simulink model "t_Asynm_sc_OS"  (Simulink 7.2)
settings: Solver=ode3  StartTime=0.0  StopTime=0.5  FixedStep=10e-6  MaxStep=1e-4  RelTol=1e-4  AbsTol=1e-4
libraries: simulink x1

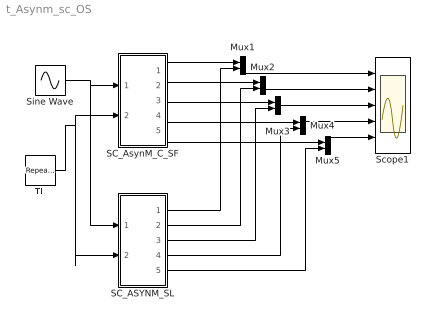
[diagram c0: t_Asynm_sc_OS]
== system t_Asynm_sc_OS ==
  Mux{1..5} (5 alike) : Mux  Inputs=2
  SC_ASYNM_SL : Subsystem  mask(SC_ASYN_MOTOR){rs=0.087, Lls=0.8e-3, rr=0.228, Llr=0.8e-3, Lm=34.7e-3, P=4, J=0.8, D=0.1, omm0=0}
      mask prompts: rs "Stator Resistance"; Lls "Stator Leakage Inductance"; rr "Rotor Resistance"; Llr "Rotor Leakage Inductance"; Lm "Magnetising Inductance"; P "Number of Poles"; J "Moment of Inertia"; D "Damping Coefficient"; omm0 "initial ang. speed"
      mask help: Open source Squirrel cage Asyn. MOTOR modeled in Simulink Blocks Input Vector u: u[0,1,2]= Three phase stator Voltages u[3]= Load Torque Output Vector y: y[0,1,2]= Three phase stator Currents y[3]= Te y[4]= Ang. Velocity W Parameter Vector p: p[0]= Rs p[1]= Ls p[2]= Rr p[3]= Lr p[4]= LM p[5]= Number of Poles P p[6]= Moment of Inertia J p[7]= Damp. Coef. D p[8]= Initial Ang. Velocity W0 You can pause the simulation during running, change the Parameters you want and continue the Simulation
  SC_AsynM_C_SF : Subsystem  mask(SC_ASYN_MOTOR){RS=0.087, LS=0.8e-3, RR=0.228, LR=0.8e-3, LM=34.7e-3, P=4, J=0.8, D=0.1, W0=0}
      mask prompts: RS "Stator Resistance"; LS "Stator Leakage Inductance"; RR "Rotor Resistance"; LR "Rotor Leakage Inductance"; LM "Magnetising Inductance"; P "Number of Poles"; J "Moment of Inertia"; D "Damping Coefficient"; W0 "initial ang. speed"
      mask help: Open source Squirrel cage Asyn. MOTOR modeled as Simulink C-S-Function Block Input Vector u: u[0,1,2]= Three phase stator Voltages u[3]= Load Torque Output Vector y: y[0,1,2]= Three phase stator Currents y[3]= Te y[4]= Ang. Velocity W Parameter Vector p: p[0]= Rs p[1]= Ls p[2]= Rr p[3]= Lr p[4]= LM p[5]= Number of Poles P p[6]= Moment of Inertia J p[7]= Damp. Coef. D p[8]= Initial Ang. Velocity W0 You can pause the simulation during running, change the Parameters you want and continue the Simulation
  Scope1 : Scope  NumInputPorts=5
  Sine Wave : Sin  Amplitude=400*sqrt(2)  Frequency=50*2*pi  Phase=[0, -2*pi/3, -4*pi/3]  SampleTime=0
  TL : simulink/Sources/Repeating Sequence  SystemSampleTime=-1  rep_seq_t="[0      0.2     0.201      0.4    0.401     1 ]"  rep_seq_y="[0       0       1000     1000   -1000   -1000]"
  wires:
  Sine Wave/1 -> SC_AsynM_C_SF/1(Vabc), SC_ASYNM_SL/1(Vabc)
  TL/1 -> SC_AsynM_C_SF/2(TL), SC_ASYNM_SL/2(Tl)
  Mux1/1 -> Scope1/1
  Mux2/1 -> Scope1/2
  Mux3/1 -> Scope1/3
  Mux4/1 -> Scope1/4
  Mux5/1 -> Scope1/5
  SC_ASYNM_SL/1(ia) -> Mux1/2
  SC_ASYNM_SL/2(ib) -> Mux2/2
  SC_ASYNM_SL/3(ic) -> Mux3/2
  SC_AsynM_C_SF/5(W) -> Mux5/1
  SC_AsynM_C_SF/1(iA) -> Mux1/1
  SC_AsynM_C_SF/2(iB) -> Mux2/1
  SC_AsynM_C_SF/3(iC) -> Mux3/1
  SC_AsynM_C_SF/4(TE) -> Mux4/1
  SC_ASYNM_SL/4(Te) -> Mux4/2
  SC_ASYNM_SL/5(w) -> Mux5/2

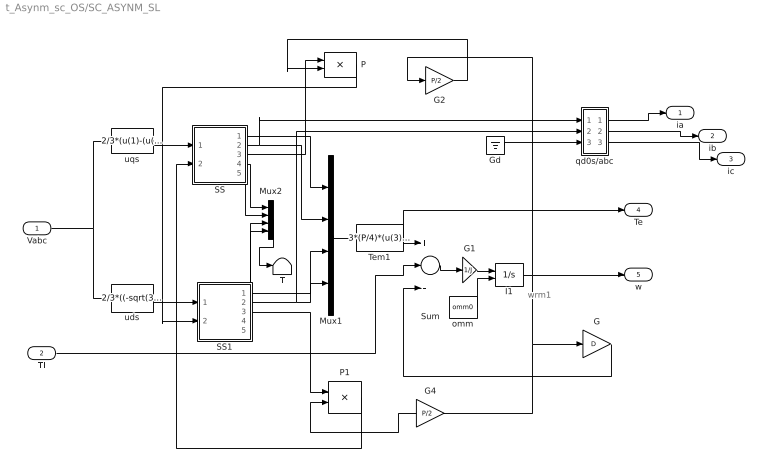
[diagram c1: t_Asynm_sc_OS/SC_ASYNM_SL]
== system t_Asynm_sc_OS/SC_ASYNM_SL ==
  note: wrm1
  Vabc : Inport
  Tl : Inport  Port=2
  G : Gain  Gain=D
  G1 : Gain  Gain=1/J
  G2 : Gain  Gain=P/2
  G4 : Gain  Gain=P/2
  Gd : Ground
  I1 : Integrator  InitialConditionSource=external
  Mux1 : Mux
  Mux2 : Mux
  P : Product
  P1 : Product
  SS : Subsystem
  SS1 : Subsystem
  Sum : Sum  Inputs=+--
  T : Terminator
  Tem1 : Fcn  Expr=3*(P/4)*(u(3)*u(2)-u(1)*u(4))
  omm : Constant  Value=omm0
  qd0s/abc : Subsystem
  uds : Fcn  Expr=2/3*((-sqrt(3)/2)*u(2)+(sqrt(3)/2)*u(3))
  uqs : Fcn  Expr=2/3*(u(1)-(u(2)/2)-(u(3)/2))
  ia : Outport
  ib : Outport  Port=2
  ic : Outport  Port=3
  Te : Outport  Port=4
  w : Outport  Port=5
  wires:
  Gd/1 -> qd0s/abc/3(0)
  SS1/1(psids) -> Mux1/3
  SS1/2(ids) -> qd0s/abc/2(d), Mux1/4
  SS1/3(psidr) -> P1/1
  SS/3(psiqr) -> P/1
  SS/1(psiqs) -> Mux1/1
  Tl/1 -> Sum/2
  Tem1/1 -> Te/1, Sum/1
  SS/2(iqs) -> qd0s/abc/1(q), Mux1/2
  G/1 -> Sum/3
  I1/1 -> w/1, G2/1, G4/1, G/1
  P/1 -> SS1/2(wr*psiqr)
  P1/1 -> SS/2(wr*psidr)
  Vabc/1 -> uds/1, uqs/1
  uds/1 -> SS1/1(uds)
  uqs/1 -> SS/1(uqs)
  G4/1 -> P1/2
  G2/1 -> P/2
  Sum/1 -> G1/1
  Mux1/1 -> Tem1/1
  SS/4(iqr) -> Mux2/1
  SS/5(psiqm) -> Mux2/2
  SS1/4(idr) -> Mux2/3
  SS1/5(psidm) -> Mux2/4
  Mux2/1 -> T/1
  G1/1 -> I1/1
  omm/1 -> I1/2
  qd0s/abc/1(a) -> ia/1
  qd0s/abc/2(b) -> ib/1
  qd0s/abc/3(c) -> ic/1

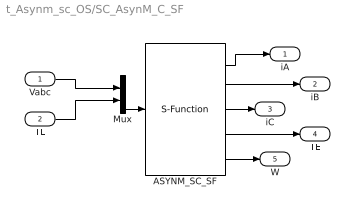
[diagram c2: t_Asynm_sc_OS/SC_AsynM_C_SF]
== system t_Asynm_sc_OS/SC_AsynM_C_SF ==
  Vabc : Inport  OutDataType=sfix(16)  OutScaling=2^0
  TL : Inport  Port=2  OutDataType=sfix(16)  OutScaling=2^0
  ASYNM_SC_SF : S-Function  FunctionName=s_Asynm_sc_OS  Parameters=[RS LS RR LR LM P J D W0]  EnableBusSupport=off
  Mux : Mux  Inputs=[3 1]
  iA : Outport  OutDataType=sfix(16)  OutScaling=2^0
  iB : Outport  Port=2  OutDataType=sfix(16)  OutScaling=2^0
  iC : Outport  Port=3  OutDataType=sfix(16)  OutScaling=2^0
  TE : Outport  Port=4  OutDataType=sfix(16)  OutScaling=2^0
  W : Outport  Port=5  OutDataType=sfix(16)  OutScaling=2^0
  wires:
  Mux/1 -> ASYNM_SC_SF/1
  Vabc/1 -> Mux/1
  TL/1 -> Mux/2
  ASYNM_SC_SF/2 -> iB/1
  ASYNM_SC_SF/3 -> iC/1
  ASYNM_SC_SF/1 -> iA/1
  ASYNM_SC_SF/4 -> TE/1
  ASYNM_SC_SF/5 -> W/1

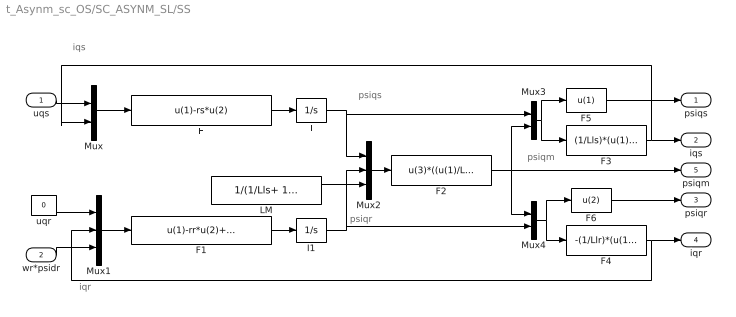
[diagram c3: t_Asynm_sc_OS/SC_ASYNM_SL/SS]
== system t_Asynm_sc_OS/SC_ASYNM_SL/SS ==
  note: iqs
  note: iqr
  note: psiqr
  note: psiqm
  note: psiqs
  uqs : Inport
  wr*psidr : Inport  Port=2
  F : Fcn  Expr=u(1)-rs*u(2)
  F1 : Fcn  Expr=u(1)-rr*u(2)+u(3)
  F2 : Fcn  Expr=u(3)*((u(1)/Lls)+(u(2)/Llr))
  F3 : Fcn  Expr=(1/Lls)*(u(1)-u(2))
  F4 : Fcn  Expr=-(1/Llr)*(u(1)-u(2))
  F5 : Fcn  Expr=u(1)
  F6 : Fcn  Expr=u(2)
  I : Integrator
  I1 : Integrator
  LM : Constant  Value=1/(1/Lls+ 1/Llr+ 1/Lm)
  Mux : Mux  Inputs=2
  Mux1 : Mux  Inputs=3
  Mux2 : Mux  Inputs=3
  Mux3 : Mux  Inputs=2
  Mux4 : Mux  Inputs=2
  uqr : Constant  Value=0
  psiqs : Outport
  iqs : Outport  Port=2
  psiqr : Outport  Port=3
  iqr : Outport  Port=4
  psiqm : Outport  Port=5
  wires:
  LM/1 -> Mux2/3
  F4/1 -> Mux1/2, iqr/1
  wr*psidr/1 -> Mux1/3
  F3/1 -> Mux/2, iqs/1
  uqr/1 -> Mux1/1
  F1/1 -> I1/1
  F6/1 -> psiqr/1
  Mux4/1 -> F6/1, F4/1
  F5/1 -> psiqs/1
  Mux3/1 -> F5/1, F3/1
  uqs/1 -> Mux/1
  I1/1 -> Mux2/2, Mux4/2
  I/1 -> Mux3/1, Mux2/1
  F2/1 -> psiqm/1, Mux4/1, Mux3/2
  Mux2/1 -> F2/1
  Mux1/1 -> F1/1
  F/1 -> I/1
  Mux/1 -> F/1

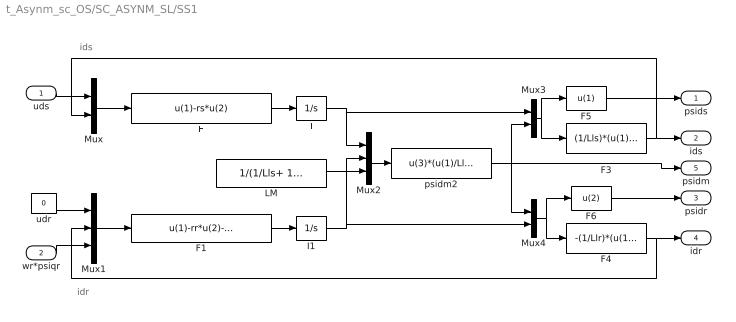
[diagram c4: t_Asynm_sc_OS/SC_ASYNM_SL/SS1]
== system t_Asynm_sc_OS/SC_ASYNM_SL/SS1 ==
  note: idr
  note: ids
  uds : Inport
  wr*psiqr : Inport  Port=2
  F : Fcn  Expr=u(1)-rs*u(2)
  F1 : Fcn  Expr=u(1)-rr*u(2)-u(3)
  F3 : Fcn  Expr=(1/Lls)*(u(1)-u(2))
  F4 : Fcn  Expr=-(1/Llr)*(u(1)-u(2))
  F5 : Fcn  Expr=u(1)
  F6 : Fcn  Expr=u(2)
  I : Integrator
  I1 : Integrator
  LM : Constant  Value=1/(1/Lls+ 1/Llr+ 1/Lm)
  Mux : Mux  Inputs=2
  Mux1 : Mux  Inputs=3
  Mux2 : Mux  Inputs=3
  Mux3 : Mux  Inputs=2
  Mux4 : Mux  Inputs=2
  psidm2 : Fcn  Expr=u(3)*(u(1)/Lls+u(2)/Llr)
  udr : Constant  Value=0
  psids : Outport
  ids : Outport  Port=2
  psidr : Outport  Port=3
  idr : Outport  Port=4
  psidm : Outport  Port=5
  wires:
  psidm2/1 -> psidm/1, Mux4/1, Mux3/2
  LM/1 -> Mux2/3
  F4/1 -> Mux1/2, idr/1
  F3/1 -> Mux/2, ids/1
  udr/1 -> Mux1/1
  wr*psiqr/1 -> Mux1/3
  F1/1 -> I1/1
  Mux/1 -> F/1
  F/1 -> I/1
  Mux1/1 -> F1/1
  Mux2/1 -> psidm2/1
  I/1 -> Mux2/1, Mux3/1
  I1/1 -> Mux2/2, Mux4/2
  uds/1 -> Mux/1
  Mux3/1 -> F3/1, F5/1
  F5/1 -> psids/1
  Mux4/1 -> F4/1, F6/1
  F6/1 -> psidr/1

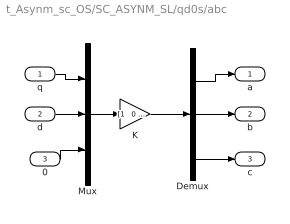
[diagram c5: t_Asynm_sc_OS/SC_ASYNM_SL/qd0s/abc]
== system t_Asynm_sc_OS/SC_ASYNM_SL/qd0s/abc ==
  q : Inport
  d : Inport  Port=2
  0 : Inport  Port=3
  Demux : Demux  Outputs=3
  K : Gain  Gain="[1   0  1;  -.5   -sqrt(3)/2   1;  -.5    sqrt(3)/2  1]"  Multiplication=Matrix(K*u)
  Mux : Mux  Inputs=3
  a : Outport
  b : Outport  Port=2
  c : Outport  Port=3
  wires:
  d/1 -> Mux/2
  K/1 -> Demux/1
  Mux/1 -> K/1
  Demux/2 -> b/1
  Demux/3 -> c/1
  0/1 -> Mux/3
  q/1 -> Mux/1
  Demux/1 -> a/1
